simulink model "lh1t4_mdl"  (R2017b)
settings: Solver=ode45  StartTime=0.0  StopTime=60.0  RelTol=1e-3  AbsTol=1e-6
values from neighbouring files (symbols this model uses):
  a1 = 1    [lh1t4_m.m]
  a2 = 1    [lh1t4_m.m]
  b1 = 0    [lh1t4_m.m]
  b2 = 0.2    [lh1t4_m.m]
  w_amplitude = 0.04    [lh1t4_m.m]
  w_delay = 4    [lh1t4_m.m]
  wz_period = 8    [lh1t4_m.m]
  x0 = 10    [lh1t4_m.m]
  x_start = 9    [lh1t4_m.m]
  y_start = 0    [lh1t4_m.m]
  z_amplitude = 2    [lh1t4_m.m]
  z_delay = 3    [lh1t4_m.m]
libraries: simulink x1

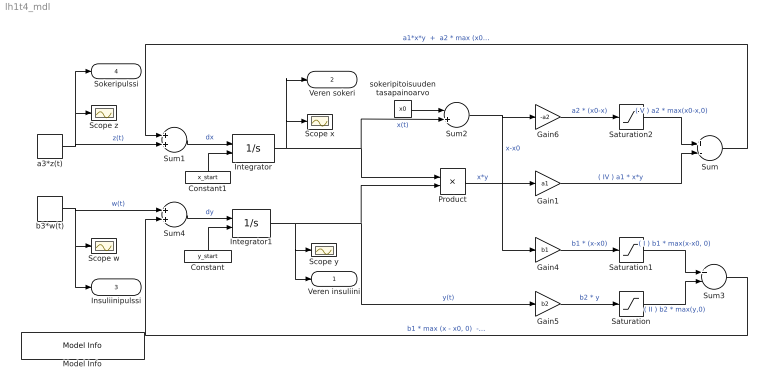
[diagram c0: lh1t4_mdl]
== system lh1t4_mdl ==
  Constant : Constant  Value=y_start
  Constant1 : Constant  Value=x_start
  Gain1 : Gain  Gain=a1
  Gain4 : Gain  Gain=b1
  Gain5 : Gain  Gain=b2
  Gain6 : Gain  Gain=-a2
  Integrator : Integrator  InitialConditionSource=external  InitialCondition=1
  Integrator1 : Integrator  InitialConditionSource=external  InitialCondition=1
  Model Info : simulink/Model-Wide Utilities/Model Info  Frame=on  DisplayStringWithTags=Laskuharjoitus 1, tehtävä 4  HorizontalTextAlignment=Center  LeftAlignmentValue=0.5
  Product : Product
  Saturation : Saturate  UpperLimit=Inf  LowerLimit=0
  Saturation1 : Saturate  UpperLimit=Inf  LowerLimit=0
  Saturation2 : Saturate  UpperLimit=Inf  LowerLimit=0
  Scope w : Scope
  Scope x : Scope
  Scope y : Scope
  Scope z : Scope
  Sum : Sum  Inputs=+-
  Sum1 : Sum
  Sum2 : Sum  Inputs=-+
  Sum3 : Sum  Inputs=+-
  Sum4 : Sum
  a3*z(t) : DiscretePulseGenerator  PulseType=Time based  Amplitude=z_amplitude  Period=wz_period  PhaseDelay=z_delay
  b3*w(t) : DiscretePulseGenerator  PulseType=Time based  Amplitude=w_amplitude  Period=wz_period  PhaseDelay=w_delay
  sokeripitoisuuden tasapainoarvo : Constant  Value=x0
  Veren insuliini : Outport
  Veren sokeri : Outport  Port=2
  Insuliinipulssi : Outport  Port=3
  Sokeripulssi : Outport  Port=4
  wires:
  b3*w(t)/1 -> Sum4/1, Insuliinipulssi/1, Scope w/1  "w(t)"
  Sum3/1 -> Sum4/2  "b1 * max (x - x0, 0)  -  b2 * max (y, 0)"
  Sum4/1 -> Integrator1/1  "dy"
  Integrator1/1 -> Product/2, Gain5/1, Scope y/1, Veren insuliini/1  "y(t)"
  Saturation2/1 -> Sum/1  "( V ) a2 * max(x0-x,0)"
  Sum2/1 -> Gain4/1, Gain6/1  "x-x0"
  Integrator/1 -> Sum2/2, Product/1, Scope x/1, Veren sokeri/1  "x(t)"
  sokeripitoisuuden tasapainoarvo/1 -> Sum2/1
  a3*z(t)/1 -> Sum1/2, Sokeripulssi/1, Scope z/1  "z(t)"
  Sum/1 -> Sum1/1  "a1*x*y  +  a2 * max (x0 - x, 0)"
  Gain1/1 -> Sum/2  "( IV ) a1 * x*y"
  Product/1 -> Gain1/1  "x*y"
  Gain6/1 -> Saturation2/1  "a2 * (x0-x)"
  Gain4/1 -> Saturation1/1  "b1 * (x-x0)"
  Saturation1/1 -> Sum3/1  "( I ) b1 * max(x-x0, 0)"
  Gain5/1 -> Saturation/1  "b2 * y"
  Saturation/1 -> Sum3/2  "( II ) b2 * max(y,0)"
  Sum1/1 -> Integrator/1  "dx"
  Constant1/1 -> Integrator/2
  Constant/1 -> Integrator1/2
